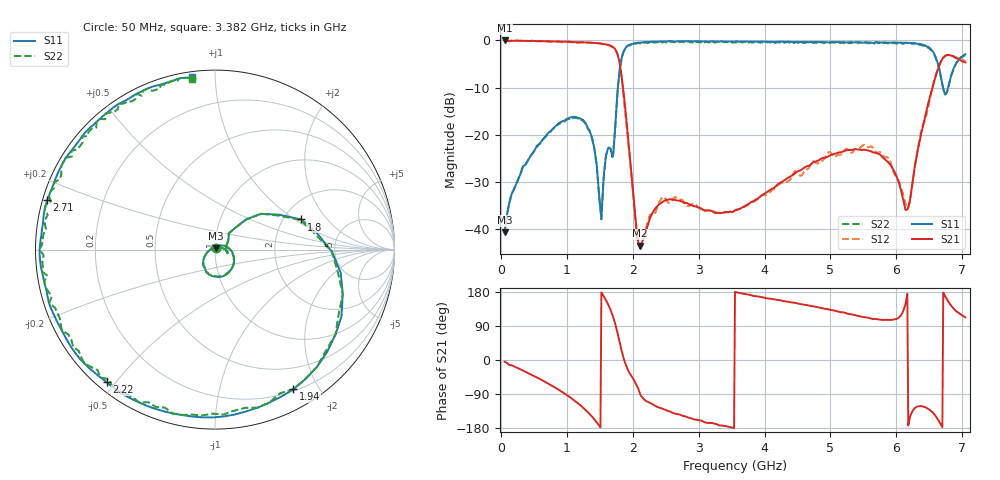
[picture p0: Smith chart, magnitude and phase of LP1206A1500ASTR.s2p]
!Instrument:	"HEWLETT PACKARD,8720ES,US39172150,7.62 "
!	LP1206	High	Performance	Low	Pass	Filters
!	P/N	LP1206A1500ASTR	6	May	2019
#	MHz	S	dB	R	50
!	Frq	S11(dB)	S11(deg)	S21(dB)	S21(deg)	S12(dB)	S12(deg)	S22(dB)	S22(deg)
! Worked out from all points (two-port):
!   501 points, 50 MHz to 7.05 GHz, reference 50 ohm
!   highest |S21| = -0.04 dB at 50 MHz (marker M1); lowest = -43.4 dB at 2.108 GHz (marker M2)
!   |S21| within 3 dB of the highest: start of sweep to 1.766 GHz
!   lowest |S11| = -40.6 dB at 50 MHz (marker M3), VSWR 1.02, Z = 50.6 + j0.737 ohm
!   |S11| at or under -10 dB: start of sweep to 1.771 GHz; 6.711 GHz to 6.787 GHz (75.88 MHz wide, 1.12 % of centre)
!   |S22| runs from -40.8 to -0.2 dB; largest |S21 - S12| = 0.053
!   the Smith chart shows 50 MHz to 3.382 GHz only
!   S11 on the Smith chart (normalised r, x): 50 MHz: 1.01, +0.01; 1.8 GHz: 2.48, +1.12; 1.94 GHz: 0.22, -1.69; 2.22 GHz: 0.03, -0.47; 2.71 GHz: 0.01, +0.14; 3.382 GHz: 0.03, +0.87
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50  -40.56 51.0  -0.04 -4.4  -0.04 -4.2  -40.76 51.0
792  -18.58 -25.6  -0.26 -70.3  -0.24 -70.5  -18.68 -25.6
1226  -16.73 -99.8  -0.42 -123.2  -0.44 -123.5  -16.93 -99.8
1520  -37.67 50.3  -0.70 178.4  -0.73 177.8  -37.87 50.3
1702  -23.75 16.3  -1.49 111.8  -1.57 110.8  -23.95 16.3
1800  -5.88 19.3  -4.92 45.1  -4.73 42.4  -5.98 19.3
1940  -0.99 -60.7  -22.80 -32.2  -23.23 -29.2  -0.99 -60.7
2108  -0.49 -107.6  -43.44 -89.5  -43.53 -84.2  -0.69 -107.6
2220  -0.41 -129.3  -39.34 -110.2  -38.56 -106.4  -0.61 -129.3
2388  -0.29 -156.2  -34.81 -125.1  -34.64 -117.3  -0.49 -156.2
2710  -0.22 163.6  -33.93 -144.1  -33.69 -145.3  -0.42 163.6
3382  -0.28 97.7  -36.39 -174.0  -36.45 -176.4  -0.38 97.7
3550  -0.30 83.2  -35.95 179.8  -36.00 177.3  -0.50 83.2
4208  -0.31 28.3  -30.37 158.3  -30.56 158.9  -0.41 28.3
4726  -0.38 -13.6  -25.94 142.0  -25.82 144.4  -0.48 -13.6
5370  -0.46 -65.9  -23.01 118.5  -23.04 125.0  -0.66 -65.9
5888  -0.50 -109.7  -25.96 105.7  -24.94 102.7  -0.50 -109.7
6182  -0.55 -137.2  -35.35 -172.7  -35.40 178.0  -0.65 -137.2
6476  -1.35 -173.9  -13.86 -128.1  -14.65 -127.7  -1.55 -173.9
6658  -6.34 156.1  -5.17 -164.5  -5.07 -166.8  -6.34 156.1
6756  -11.13 -171.3  -3.21 164.2  -3.21 162.5  -11.33 -171.3
7050  -2.94 -173.1  -4.69 112.7  -4.39 112.2  -3.04 -173.1
